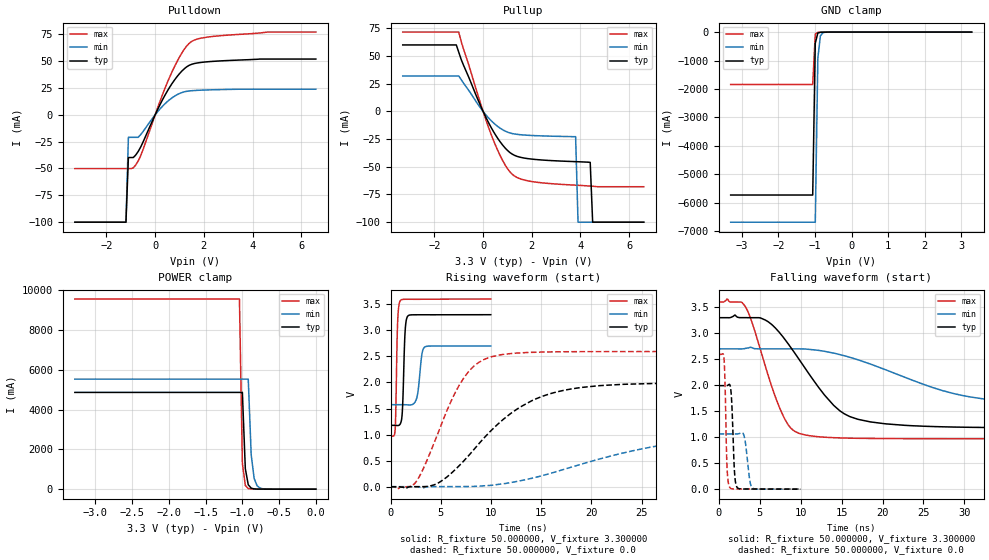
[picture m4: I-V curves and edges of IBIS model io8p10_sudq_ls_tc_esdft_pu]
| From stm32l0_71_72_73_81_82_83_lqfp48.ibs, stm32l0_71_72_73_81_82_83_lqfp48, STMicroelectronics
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|   Model io8p10_sudq_ls_tc_esdft_pu
[Model]  io8p10_sudq_ls_tc_esdft_pu
Model_type I/O
Polarity   Non-Inverting
Enable   Active-Low
Vinl =   0.990000V
Vinh =   2.310000V
Vmeas =  1.650000V
Cref =   50.000000pF
Rref =   100.000000M
Vref =   0.0V
C_comp   2.248300pF   2.207300pF   2.311900pF
[Temperature Range]   25.000000   0.125000k   -40.000000
[Pullup Reference]   3.300000V   2.700000V   3.600000V
[Pulldown Reference]   0.0V   0.0V   0.0V
[POWER Clamp Reference]   3.300000V   2.700000V   3.600000V
[GND Clamp Reference]   0.0V   0.0V   0.0V
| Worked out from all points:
|   slope of the pulldown table from 0 to 0.495 V, typ, clamps not added: 22.6 ohm
|   slope of the pullup table from 0 to 0.495 V, typ, clamps not added: 23.9 ohm
|   GND clamp passes 1 mA (typ) near -0.64 V on its own axis
|   POWER clamp passes 1 mA (typ) near -0.63 V on its own axis
|   rising waveform, R_fixture 50.000000, V_fixture 3.300000: 20-80 % time 208ps typ, 362ps min, 164ps max; typ from 1.18 V to 3.3 V
|   rising waveform, R_fixture 50.000000, V_fixture 0.0: 20-80 % time 6.73ns typ, 13.7ns min, 3.61ns max; typ from 0.001 V to 1.99 V
|   falling waveform, R_fixture 50.000000, V_fixture 3.300000: 20-80 % time 6ns typ, 12.6ns min, 3.28ns max; typ from 3.3 V to 1.18 V
|   falling waveform, R_fixture 50.000000, V_fixture 0.0: 20-80 % time 290ps typ, 459ps min, 228ps max; typ from 1.99 V to 0.001 V
[Pulldown]
|Voltage   I(typ)   I(min)   I(max)
-3.3V     -100mA     -100mA     -50.11mA
-1.2V     -100mA     -100mA     -50.11mA
-1.1V     -39.8mA    -21mA      -50.11mA
-900mV    -39.8mA    -21mA      -49.43mA
-600mV    -30.26mA   -18.59mA   -38.38mA
500mV     22.11mA    12.28mA    30.06mA
900mV     35.58mA    18.71mA    49.62mA
1.3V      44.74mA    21.88mA    64.23mA
1.7V      48.13mA    22.72mA    70.3mA
2.4V      49.79mA    23.31mA    73.03mA
4.6V      51.9mA     23.82mA    77mA
6.6V      51.9mA     23.82mA    77mA
[Pullup]
|Voltage   I(typ)   I(min)   I(max)
-3.3V     60mA       32mA       71.6mA
-1.1V     60mA       32mA       71.6mA
-1V       53.5mA     32mA       71.6mA
-100mV    4.893mA    2.926mA    6.861mA
400mV     -17.21mA   -9.813mA   -24.69mA
900mV     -32.92mA   -17.72mA   -48.15mA
1.3V      -39.75mA   -20.41mA   -58.47mA
3.8V      -45.36mA   -22.8mA    -66.6mA
3.9V      -45.44mA   -100mA     -66.72mA
4.4V      -46mA      -100mA     -67.4mA
4.5V      -100mA     -100mA     -67.56mA
6.6V      -100mA     -100mA     -68mA
[GND_clamp]
|Voltage   I(typ)   I(min)   I(max)
-3.3V     -5.732A    -6.688A    -1.842A
-1.06V    -5.732A    -6.688A    -1.842A
-990mV    -389.4mA   -6.688A    -68.34mA
-920mV    -32.57mA   -918.2mA   -10.72mA
-850mV    -6.763mA   -131mA     -6.509mA
-780mV    -3.471mA   -21mA      -4.208mA
3.28V     0A         0A         0A
[POWER_clamp]
|Voltage   I(typ)   I(min)   I(max)
-3.28V    4.87A      5.538A     9.569A
-1.04V    4.87A      5.538A     9.569A
-1V       4.87A      5.538A     1.315A
-960mV    1.032A     5.538A     186.5mA
-920mV    222.2mA    5.538A     31.65mA
-880mV    50.75mA    1.734A     9.59mA
-840mV    13.94mA    544.9mA    5.676mA
-800mV    5.568mA    172.7mA    4.284mA
-760mV    3.243mA    55.85mA    3.306mA
-680mV    1.609mA    7mA        1.749mA
0V        0A         0A         0A
[Ramp]
| variable   typ   min   max
dV/dt_r  1.19491/6.72069n   0.62752/13.71273n   1.55546/3.60216n
dV/dt_f  1.27284/5.99337n   0.65196/12.48544n   1.57747/3.27738n
R_load = 50.000000
[Rising Waveform]
R_fixture= 50.000000
V_fixture= 3.300000
V_fixture_min= 2.700000
V_fixture_max= 3.600000
|time   V(typ)   V(min)   V(max)
0s        1.178V     1.575V     970.9mV
440.4ps   1.177V     1.575V     1.086V
680.7ps   1.174V     1.575V     3.099V
961ps     1.208V     1.575V     3.57V
1.181ns   1.519V     1.575V     3.593V
1.441ns   2.993V     1.574V     3.596V
1.702ns   3.273V     1.571V     3.596V
2.603ns   3.299V     1.708V     3.595V
3.423ns   3.299V     2.684V     3.597V
9.97ns    3.3V       2.7V       3.6V
[Rising Waveform]
R_fixture= 50.000000
V_fixture= 0.0
V_fixture_min= 0.0
V_fixture_max= 0.0
|time   V(typ)   V(min)   V(max)
0s        1.083mV    1.822mV    1.032mV
2.503ns   2.348mV    -1.697mV   88.4mV
4.705ns   70.57mV    3.968mV    1.024V
6.907ns   420.2mV    4.128mV    1.972V
8.308ns   717.7mV    6.925mV    2.316V
10.01ns   1.078V     27.49mV    2.492V
14.11ns   1.655V     165.1mV    2.578V
19.02ns   1.905V     434.3mV    2.592V
31.83ns   1.99V      922.1mV    2.593V
49.85ns   1.993V     1.064V     2.593V
[Falling Waveform]
R_fixture= 50.000000
V_fixture= 3.300000
V_fixture_min= 2.700000
V_fixture_max= 3.600000
|time   V(typ)   V(min)   V(max)
0s        3.3V       2.7V       3.6V
3.303ns   3.3V       2.71V      3.502V
5.706ns   3.254V     2.7V       2.365V
7.508ns   2.998V     2.7V       1.542V
8.609ns   2.771V     2.7V       1.214V
9.81ns    2.5V       2.7V       1.076V
14.01ns   1.618V     2.619V     991.9mV
17.02ns   1.344V     2.489V     979.5mV
30.73ns   1.191V     1.774V     971.2mV
49.85ns   1.178V     1.575V     970.9mV
[Falling Waveform]
R_fixture= 50.000000
V_fixture= 0.0
V_fixture_min= 0.0
V_fixture_max= 0.0
|time   V(typ)   V(min)   V(max)
0s        1.993V     1.064V     2.593V
660.7ps   1.993V     1.064V     2.515V
1.021ns   1.994V     1.064V     453.5mV
1.341ns   2.015V     1.064V     40.7mV
1.582ns   1.725V     1.064V     10.37mV
1.962ns   280mV      1.064V     5.232mV
2.282ns   29.76mV    1.064V     5.004mV
3.103ns   3.944mV    1.029V     5.119mV
4.124ns   3.927mV    23.57mV    4.533mV
9.97ns    1.083mV    1.822mV    1.032mV
